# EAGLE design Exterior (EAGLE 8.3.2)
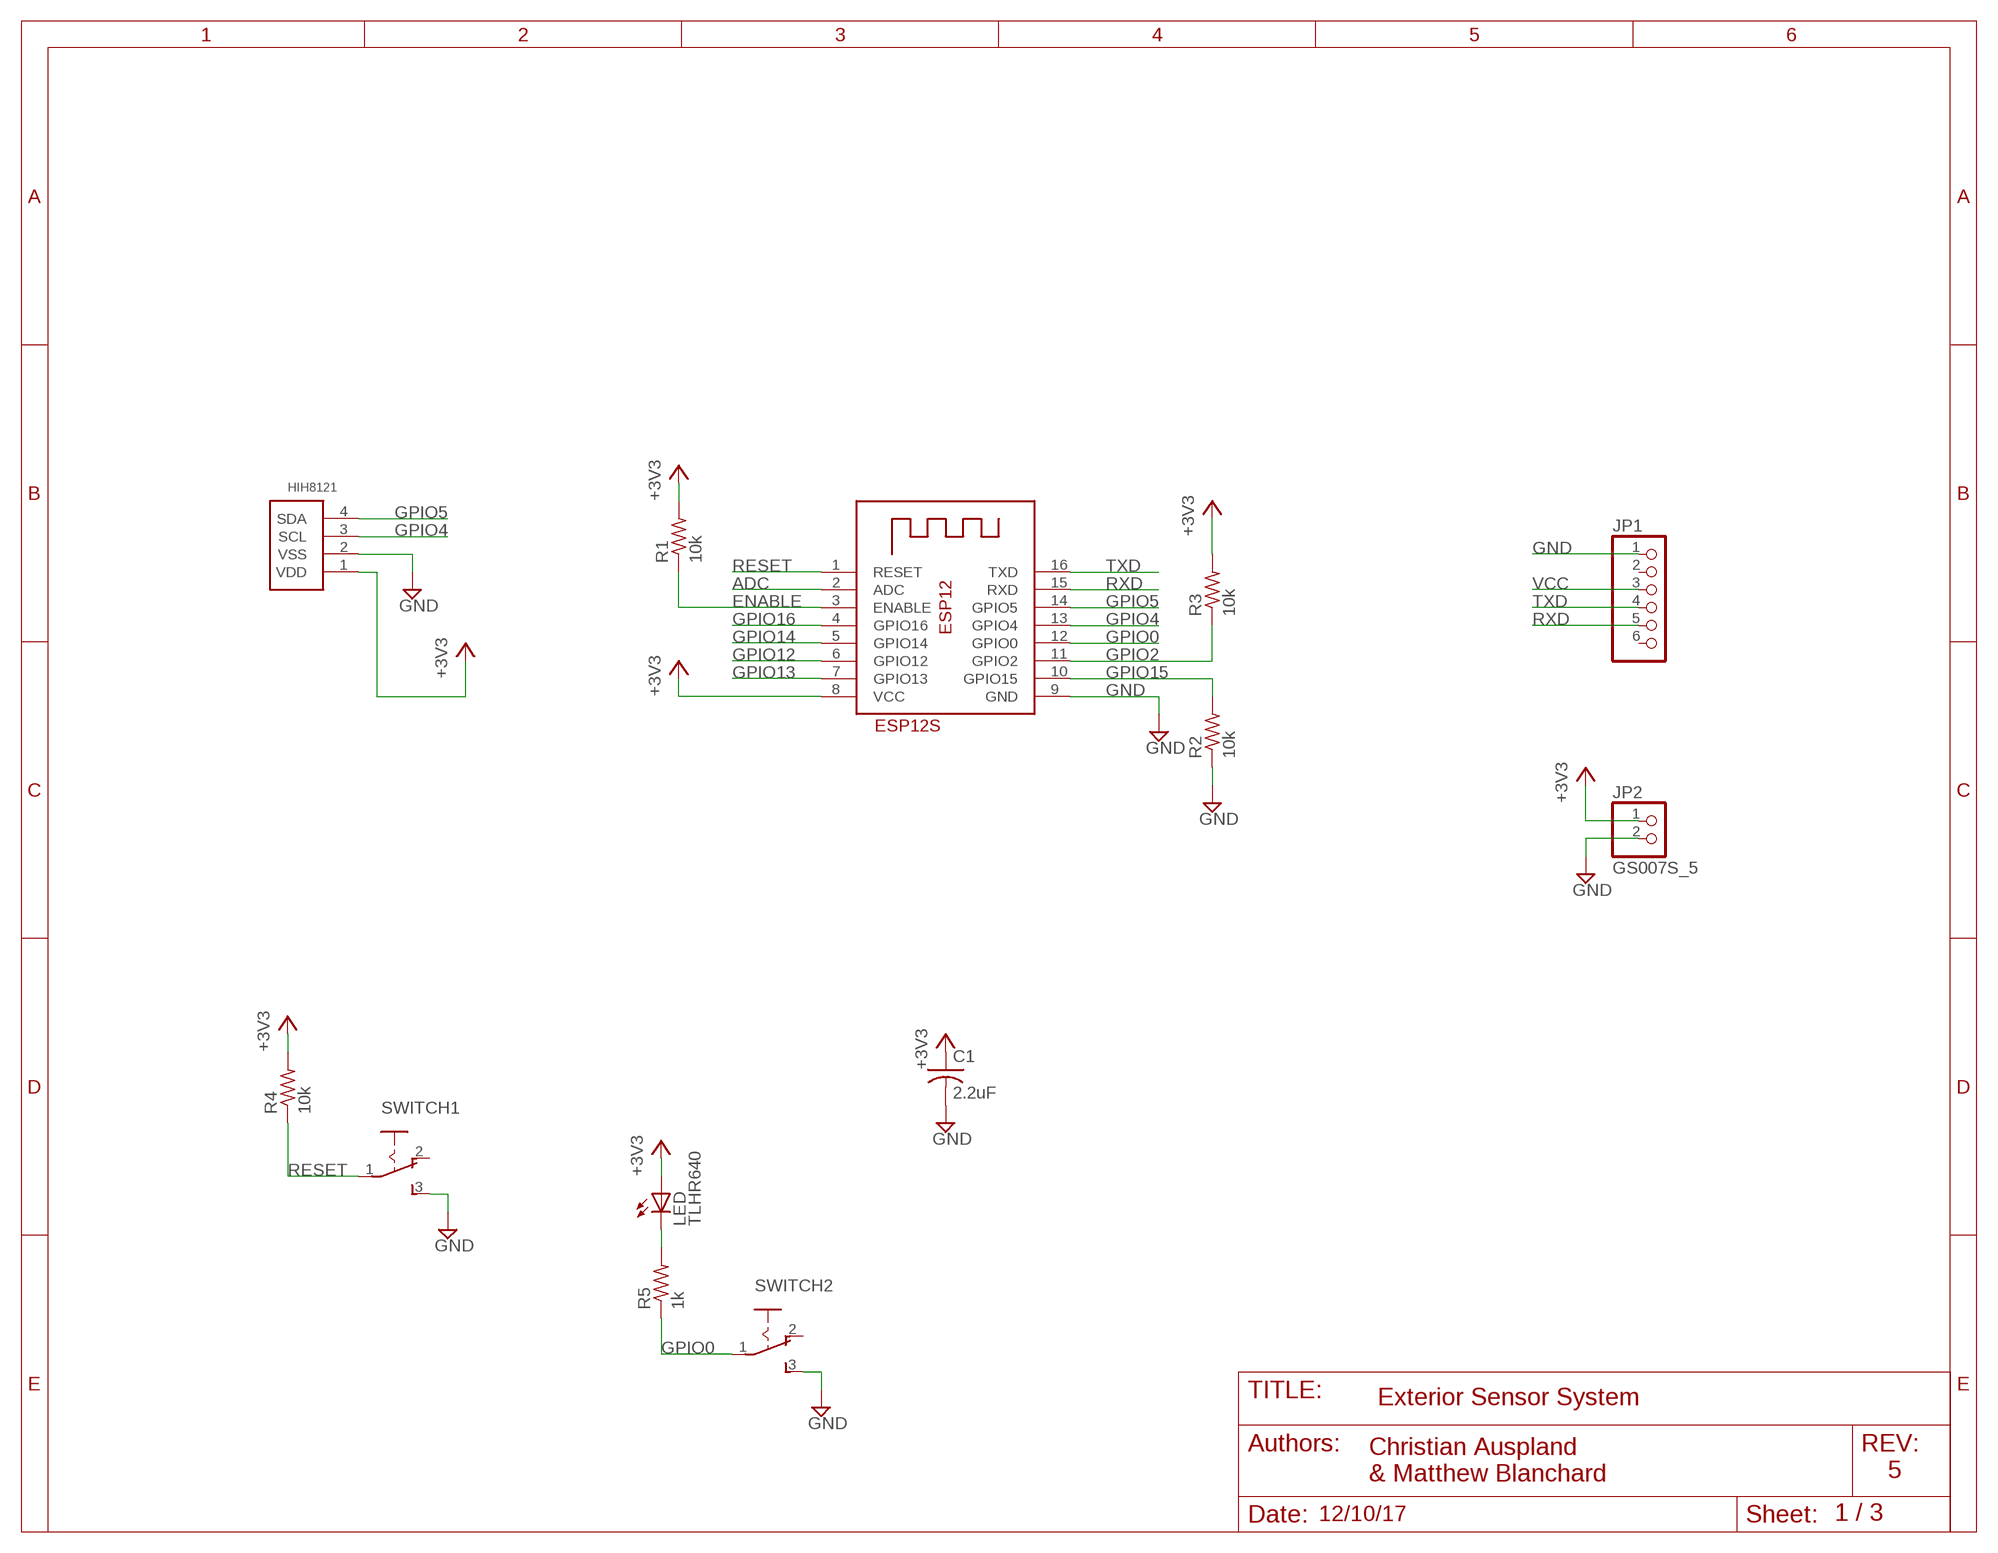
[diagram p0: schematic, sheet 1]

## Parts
C1  2.2uF  UMA1V2R2MCD2TP  [UMA1V2R2MCD2TP]
ESP12S  MYESP12S  [MYESP12S]
HIH8121  HIH8121  [HIH8121]
JP1  PINHD-1X6  [1X06]
JP2  GS007S_5  [GS007S_5]
LED  TLHR640  [TLHR640]
R1  10k  R10K  [R10K]
R2  10k  R10K  [R10K]
R3  10k  R10K  [R10K]
R4  10k  R10K  [R10K]
R5  1k  R10K  [R10K]
SWITCH1  URBEST11863  [URBEST11863]
SWITCH2  URBEST11863  [URBEST11863]

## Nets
+3V3: C1.A ESP12S.8(VCC) HIH8121.1(VDD) JP2.1 LED.A R1.2 R3.2 R4.2
ADC: ESP12S.2(ADC)
ENABLE: ESP12S.3(ENABLE) R1.1
GND: C1.C ESP12S.9(GND) HIH8121.2(VSS) JP1.1 JP2.2 R2.1 SWITCH1.3(GND) SWITCH2.3(GND)
GPIO0: ESP12S.12(GPIO0) R5.1 SWITCH2.1(RESET)
GPIO2: ESP12S.11(GPIO2) R3.1
GPIO4: ESP12S.13(GPIO4) HIH8121.3(SCL)
GPIO5: ESP12S.14(GPIO5) HIH8121.4(SDA)
GPIO12: ESP12S.6(GPIO12)
GPIO13: ESP12S.7(GPIO13)
GPIO14: ESP12S.5(GPIO14)
GPIO15: ESP12S.10(GPIO15) R2.2
GPIO16: ESP12S.4(GPIO16)
N$1: LED.C R5.2
RESET: ESP12S.1(RESET) R4.1 SWITCH1.1(RESET)
RXD: ESP12S.15(RXD) JP1.5
TXD: ESP12S.16(TXD) JP1.4
VCC: JP1.3
Unconnected: JP1.2 JP1.6 SWITCH1.2(VCC) SWITCH2.2(VCC)

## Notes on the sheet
- Exterior Sensor System
- 5
- Christian Auspland
  & Matthew Blanchard
- 12/10/17 | 1 / 3

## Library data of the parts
C1 = MyLibrary:UMA1V2R2MCD2TP
ESP12S = MyLibrary:MYESP12S
HIH8121 = MyLibrary:HIH8121
JP1 = adafruit:PINHD-1X6: PIN HEADER
JP2 = MyLibrary:GS007S_5
LED = MyLibrary:TLHR640
R1-R5 = MyLibrary:R10K
SWITCH1 SWITCH2 = MyLibrary:URBEST11863

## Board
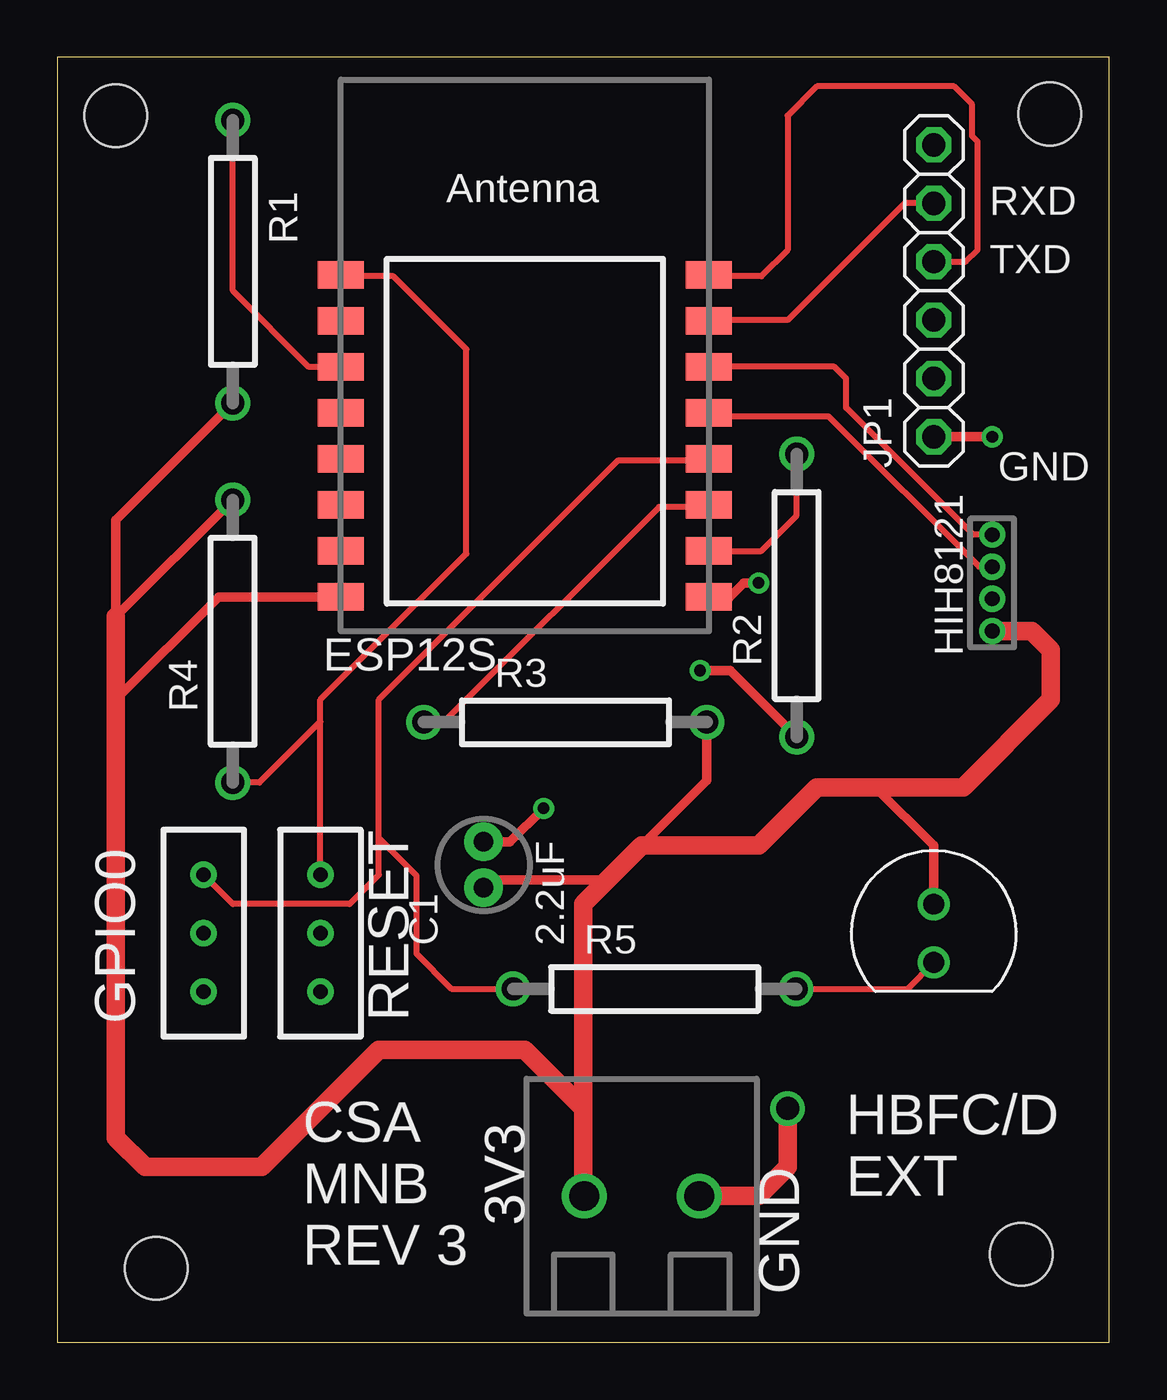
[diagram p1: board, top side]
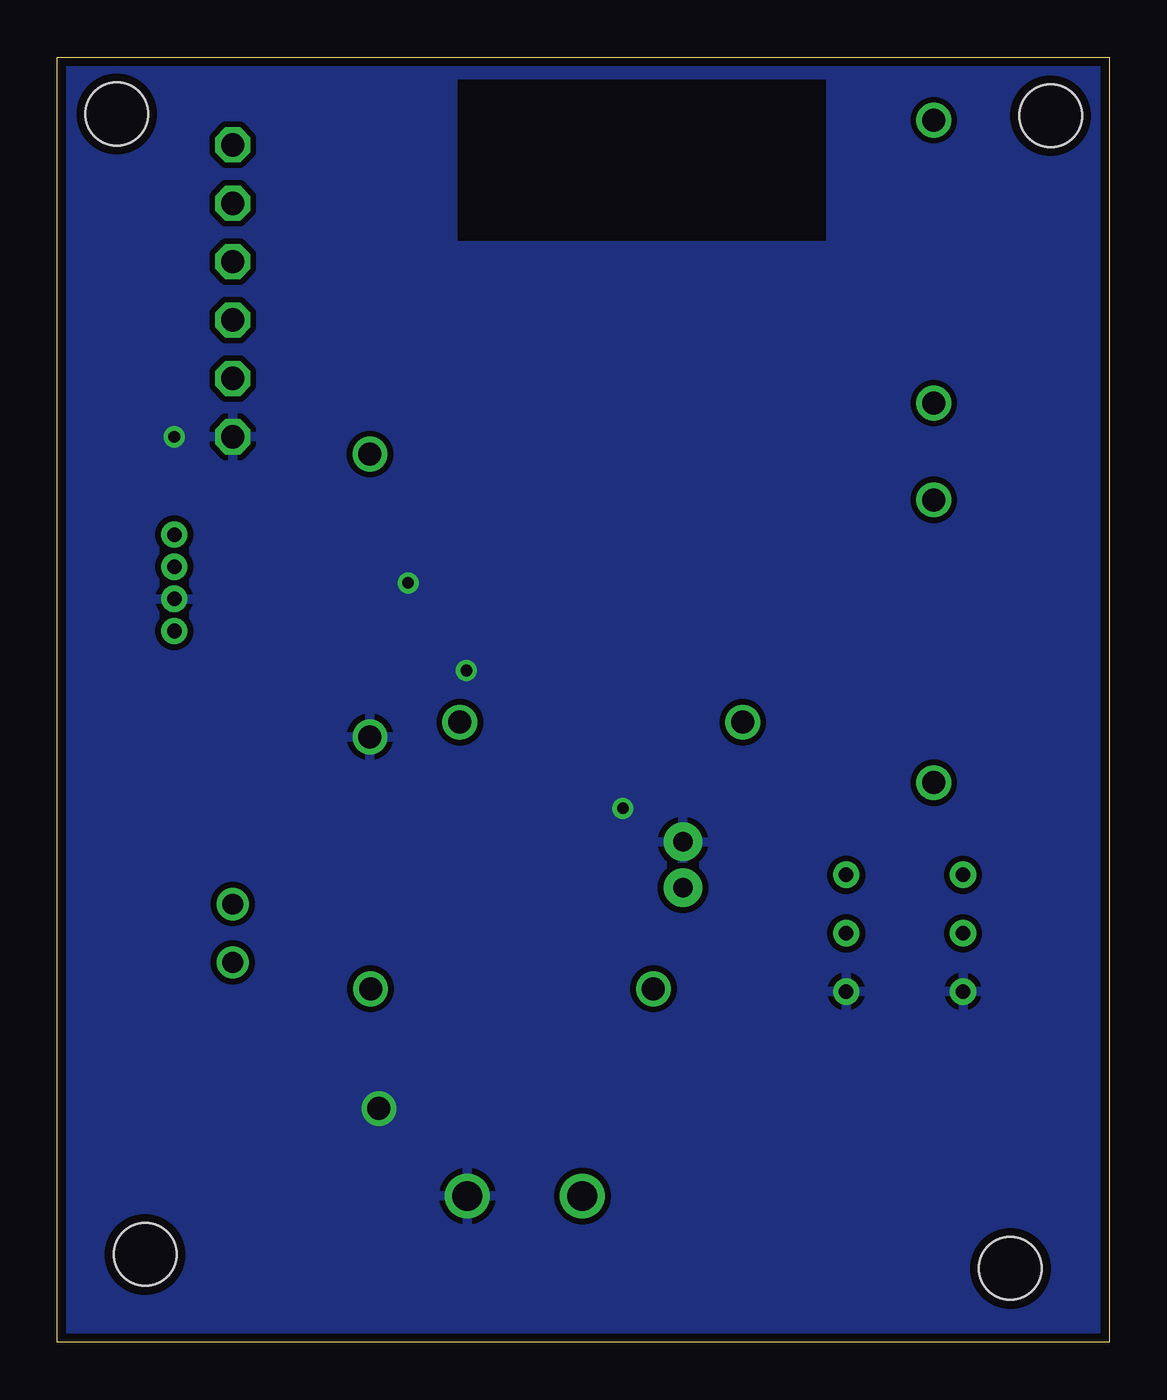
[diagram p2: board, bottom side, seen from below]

Size 45.72 x 55.87 mm. Coordinates in mm from the lower left corner, seen from the top.
Outline: 0,0 45.72,0 45.72,55.87 0,55.87 0,0
Copper layers (1*16): Top 0.035mm / dielectric 1.5mm / Bottom 0.035mm
Design rules "default *": minimum track width 10mil, minimum drill 15mil, track to track 10mil, track to pad 10mil, pad to pad 10mil, via to via 10mil, smd to smd 6mil, copper to edge 15mil, drill to drill 10mil, minimum pad ring 10mil, minimum via ring 8mil, stop-mask expansion 4mil, vias tented up to drill 0mil, thermal gap 10mil
Holes 2.73 mm at 2.54,53.34 4.29,3.2 41.91,3.81 43.14,53.42

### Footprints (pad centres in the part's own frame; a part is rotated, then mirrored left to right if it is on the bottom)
UMA1V2R2MCD2TP = drill 0.85 pad 1.676: A -1,0; C 1,0
MYESP12S = smd 2 x 1.2: 1 -8,4.5; 2 -8,2.5; 3 -8,0.5; 4 -8,-1.5; 5 -8,-3.5; 6 -8,-5.5; 7 -8,-7.5; 8 -8,-9.5; 9 8,-9.5; 10 8,-7.5; 11 8,-5.5; 12 8,-3.5; 13 8,-1.5; 14 8,0.5; 15 8,2.5; 16 8,4.5
HIH8121 = drill 0.635 pad 1.016: 1 -2.095,0; 2 -0.699,0; 3 0.699,0; 4 2.095,0
1X06 = drill 1.016 octagon: 1 -6.35,0; 2 -3.81,0; 3 -1.27,0; 4 1.27,0; 5 3.81,0; 6 6.35,0
GS007S_5 = drill 1.3: 1 -2.5,0; 2 2.5,0
TLHR640 = drill 0.9: A -1.27,0; C 1.27,0
R10K = drill 1: 1 -6.15,0; 2 6.15,0
URBEST11863 = drill 0.635 pad 1.016: 1 -2.54,0; 2 0,0; 3 2.54,0

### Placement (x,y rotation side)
C1  18.53,20.75 90 top
ESP12S  20.32,41.91 0 top
HIH8121  40.64,33.02 90 top
JP1  38.1,45.72 90 top
JP2  25.4,6.35 0 top
LED  38.1,17.78 270 top
R1  7.62,46.99 270 top
R2  32.14,32.47 90 top
R3  22.08,26.96 0 top
R4  7.62,30.48 90 top
R5  25.96,15.36 0 top
SWITCH1  11.43,17.78 270 top
SWITCH2  6.35,17.78 270 top

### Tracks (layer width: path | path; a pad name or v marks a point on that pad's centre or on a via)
+3V3
  Top 0.406: 35.56,24.13 38.1,21.59 LED.A | 23.9,20.09 18.86,20.09 C1.A | R4.2 2.54,31.55 2.54,35.76 R1.2 | ESP12S.8 7.01,32.41 2.54,27.94 | 25.4,21.59 28.23,24.42 R3.2
  Top 0.813: JP2.1 22.86,6.39 22.86,10.16 | 22.86,10.16 22.86,19.05 23.9,20.09 25.4,21.59 30.48,21.59 33.02,24.13 35.56,24.13 39.37,24.13 43.18,27.94 43.18,30.1 42.35,30.92 HIH8121.1 | 22.86,10.16 20.32,12.7 13.97,12.7 8.89,7.62 3.81,7.62 2.54,8.89 2.54,27.94 2.54,31.55
ENABLE
  Top 0.254: ESP12S.3 10.93,42.41 7.62,45.72 R1.1
GND  (via drill 0.51, 1)
  Top 0.406: v30.48,33.02 29.84,33.02 29.21,32.39 28.34,32.39 ESP12S.9 | v40.64,39.37 JP1.1 | C1.C 19.67,21.75 v21.13,23.22 | R2.1 29.25,29.21 v27.94,29.21
  Top 0.813: v31.75,10.16 31.75,7.62 30.48,6.35 JP2.2
  pour Bottom: 0,55.88 44.45,55.88 45.72,55.88 45.72,0 0,0
GPIO0
  Top 0.254: ESP12S.12 28.26,38.35 24.38,38.35 13.97,27.94 13.97,21.93 | 13.97,21.93 13.97,20.32 12.7,19.05 7.62,19.05 SWITCH2.1 | 13.97,21.93 15.61,20.29 15.61,16.89 17.13,15.37 R5.1
GPIO2
  Top 0.254: ESP12S.11 28.23,36.32 26.16,36.32 16.8,26.96 R3.1
GPIO4
  Top 0.254: ESP12S.13 28.47,40.26 33.53,40.26 40.07,33.72 HIH8121.3
GPIO5
  Top 0.254: ESP12S.14 33.78,42.42 34.29,41.91 34.29,40.64 39.82,35.11 HIH8121.4
GPIO15
  Top 0.254: ESP12S.10 30.6,34.41 32.14,35.95 R2.2
N$1
  Top 0.254: R5.2 36.96,15.37 LED.C
RESET
  Top 0.254: SWITCH1.1 11.43,26.99 | 11.43,26.99 11.43,27.94 17.78,34.29 17.78,43.18 14.61,46.36 12.38,46.36 ESP12S.1 | 11.43,26.99 8.77,24.33 R4.1
RXD
  Top 0.254: JP1.5 36.83,49.53 31.75,44.45 28.36,44.45 ESP12S.15
TXD
  Top 0.254: JP1.4 39.5,46.99 40.01,47.5 40.01,52.21 39.77,52.45 39.77,53.83 38.99,54.61 33.02,54.61 31.75,53.34 31.75,47.5 30.61,46.36 28.38,46.36 ESP12S.16

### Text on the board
tPlace: RXD | GPIO0 | RESET | GND | 3V3 | CSA / MNB / REV 3
tNames: TXD | GND | HBFC/D / EXT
